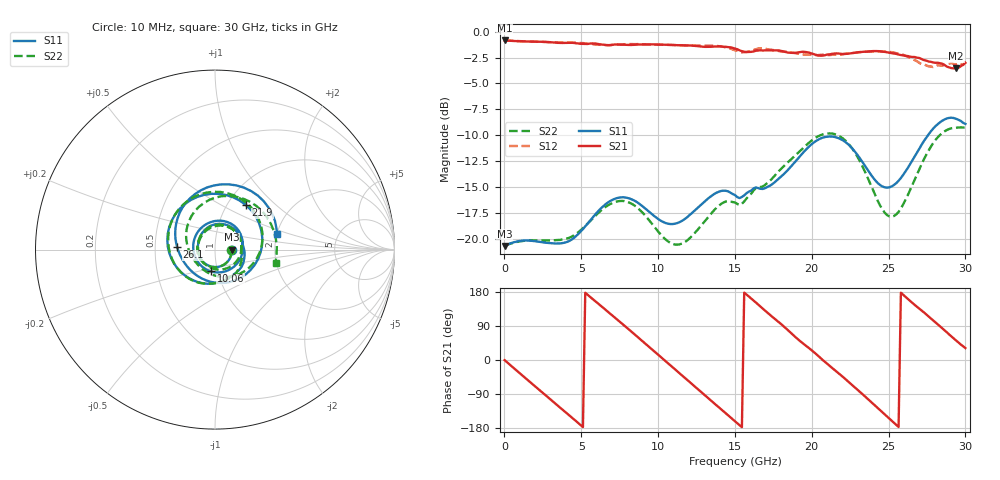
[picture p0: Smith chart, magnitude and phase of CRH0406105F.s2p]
#HZ S MA R 50
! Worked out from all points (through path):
!   201 points, 10 MHz to 30 GHz, reference 50 ohm
!   highest |S21| = -0.84 dB at 10 MHz (marker M1); lowest = -3.5 dB at 29.4 GHz (marker M2)
!   group delay of S21, straight-line fit = 97.1 ps
!   lowest |S11| = -20.7 dB at 10 MHz (marker M3), VSWR 1.20, Z = 60.1 - j0.054 ohm
!   |S11| at or under -10 dB: start of sweep to 27.57 GHz
!   |S22| runs from -20.7 to -9.2 dB; largest |S21 - S12| = 0.049
!   S11 on the Smith chart (normalised r, x): 10 MHz: 1.20, -0.00; 10.06 GHz: 0.93, -0.23; 21.9 GHz: 1.22, +0.66; 26.1 GHz: 0.65, +0.02; 30 GHz: 2.01, +0.40
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1e7  0.09203 -0.3  0.9082 -0.4  0.9079 -0.4  0.09182 -0.2
1.35955e9  0.09782 -63.1  0.8978 -47.6  0.8995 -47.4  0.09763 -62.6
2.55915e9  0.09571 -122.0  0.8948 -88.9  0.8927 -88.9  0.09779 -121.5
3.75875e9  0.09499 -174.7  0.8832 -130.3  0.8884 -130.3  0.09885 -176.0
5.1083e9  0.111 -223.3  0.8745 -177.0  0.8821 -176.5  0.1121 -226.2
6.15795e9  0.137 -263.4  0.8709 -213.1  0.8657 -213.3  0.134 -265.2
7.65745e9  0.1583 -331.0  0.8662 -264.2  0.8681 -265.0  0.152 -329.5
8.7071e9  0.1485 -384.5  0.8686 -300.7  0.8729 -300.5  0.1398 -381.0
1.005665e10  0.1235 -460.6  0.8677 -347.9  0.866 -348.1  0.1069 -456.2
1.125625e10  0.1188 -528.8  0.8617 -390.0  0.8619 -390.1  0.09335 -526.9
1.275575e10  0.1449 -601.0  0.8491 -442.5  0.8573 -442.9  0.1144 -601.0
1.5005e10  0.1622 -700.3  0.8292 -521.6  0.8139 -521.9  0.1494 -707.8
1.635455e10  0.1766 -753.2  0.8094 -567.8  0.8228 -568.5  0.1753 -767.6
1.77041e10  0.1905 -815.1  0.814 -615.1  0.8098 -614.9  0.2059 -836.5
2.01033e10  0.2902 -933.6  0.7812 -697.8  0.7726 -699.0  0.3021 -948.0
2.19027e10  0.3021 -1024.8  0.782 -760.1  0.7765 -760.1  0.3095 -1030.5
2.355215e10  0.2196 -1119.5  0.803 -819.3  0.8009 -819.1  0.2036 -1116.2
2.505165e10  0.1768 -1212.7  0.792 -874.6  0.7998 -875.3  0.1279 -1208.9
2.61013e10  0.2112 -1263.4  0.7647 -913.4  0.7654 -912.6  0.1538 -1266.7
2.775075e10  0.3297 -1330.7  0.716 -970.1  0.6794 -970.7  0.278 -1343.1
2.94002e10  0.3792 -1401.7  0.6654 -1028.9  0.6958 -1026.0  0.3438 -1422.8
3e10  0.3584 -1425.9  0.7073 -1048.4  0.7185 -1047.8  0.3452 -1452.2
